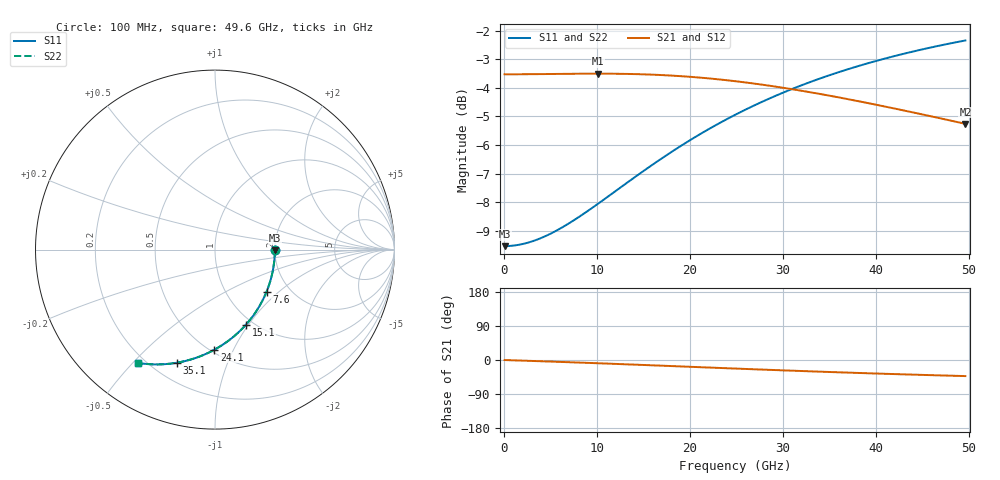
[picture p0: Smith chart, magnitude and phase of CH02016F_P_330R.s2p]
# GHz S RI R 330
! S-Parameters data
! Freq  reS11  imS11  reS21  imS21  reS12  imS12  reS22  imS22
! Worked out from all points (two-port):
!   100 points, 100 MHz to 49.6 GHz, reference 330 ohm
!   highest |S21| = -3.50 dB at 10.1 GHz (marker M1); lowest = -5.3 dB at 49.6 GHz (marker M2)
!   |S21| within 3 dB of the highest: start of sweep to end of sweep
!   lowest |S11| = -9.5 dB at 100 MHz (marker M3), VSWR 2.00, Z = 660 - j4.75 ohm
!   |S11| at or under -10 dB: nowhere
!   |S22| runs from -9.5 to -2.3 dB; largest |S21 - S12| = 0
!   S11 on the Smith chart (normalised r, x): 100 MHz: 2.00, -0.01; 7.6 GHz: 1.53, -0.83; 15.1 GHz: 0.93, -0.97; 24.1 GHz: 0.52, -0.85; 35.1 GHz: 0.30, -0.68; 49.6 GHz: 0.17, -0.52
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0.1  0.3333 -0.0032  0.6667 -0.000947  0.6667 -0.000947  0.3333 -0.0032
1.6  0.3312 -0.0511  0.6666 -0.0152  0.6666 -0.0152  0.3312 -0.0511
3.6  0.3227 -0.1142  0.6662 -0.0343  0.6662 -0.0343  0.3227 -0.1142
5.6  0.308 -0.1753  0.6654 -0.0538  0.6654 -0.0538  0.308 -0.1753
7.6  0.2876 -0.2338  0.664 -0.0738  0.664 -0.0738  0.2876 -0.2338
8.6  0.2755 -0.2617  0.6629 -0.084  0.6629 -0.084  0.2755 -0.2617
10.1  0.2551 -0.3018  0.6609 -0.0994  0.6609 -0.0994  0.2551 -0.3018
12.6  0.2163 -0.3634  0.656 -0.1257  0.656 -0.1257  0.2163 -0.3634
15.1  0.1726 -0.4181  0.6488 -0.1522  0.6488 -0.1522  0.1726 -0.4181
16.6  0.1447 -0.4475  0.6434 -0.168  0.6434 -0.168  0.1447 -0.4475
18.1  0.1159 -0.4743  0.6372 -0.1836  0.6372 -0.1836  0.1159 -0.4743
20.1  0.0766 -0.5063  0.6274 -0.2039  0.6274 -0.2039  0.0766 -0.5063
22.1  0.0366 -0.534  0.6163 -0.2234  0.6163 -0.2234  0.0366 -0.534
24.1  -0.00343 -0.5577  0.6038 -0.242  0.6038 -0.242  -0.00343 -0.5577
25.1  -0.0234 -0.5682  0.5971 -0.2508  0.5971 -0.2508  -0.0234 -0.5682
29.1  -0.1018 -0.6016  0.568 -0.2831  0.568 -0.2831  -0.1018 -0.6016
33.1  -0.1767 -0.6231  0.5363 -0.31  0.5363 -0.31  -0.1767 -0.6231
35.1  -0.2123 -0.6302  0.5198 -0.3214  0.5198 -0.3214  -0.2123 -0.6302
38.1  -0.2634 -0.6369  0.4949 -0.336  0.4949 -0.336  -0.2634 -0.6369
41.6  -0.3191 -0.6396  0.4659 -0.3495  0.4659 -0.3495  -0.3191 -0.6396
45.6  -0.3776 -0.6375  0.4336 -0.3609  0.4336 -0.3609  -0.3776 -0.6375
49.6  -0.4308 -0.6311  0.4028 -0.3685  0.4028 -0.3685  -0.4308 -0.6311
